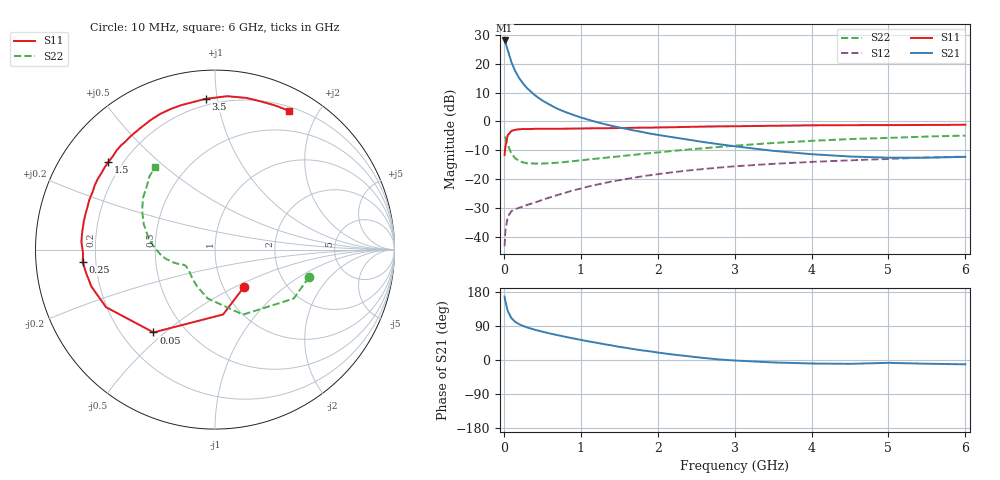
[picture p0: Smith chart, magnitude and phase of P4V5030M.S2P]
! SIEMENS Small Signal Semiconductors
! BFP182
! Si NPN RF Bipolar Junction Transistor in SOT143
! VCE = 0.5 V  IC = 30 mA
! Common Emitter S-Parameters:  March  1996
# GHz  S  MA  R  50
!  f  S11  S21  S12  S22
! GHz  MAG  ANG  MAG  ANG  MAG  ANG  MAG  ANG
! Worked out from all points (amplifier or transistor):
!   36 points, 10 MHz to 6 GHz, reference 50 ohm
!   highest |S21| = 28.2 dB at 10 MHz (marker M1)
!   |S21| within 3 dB of that: start of sweep to 46.69 MHz
!   unconditionally stable (mu >= 1): start of sweep to 23.08 MHz; 140.7 MHz to end of sweep
!   at 250 MHz: K = 1.46, MAG = 17.4 dB, |S12| = -29.6 dB
!   at 1.4 GHz: K = 2.64, MAG = 2.6 dB, |S12| = -20.9 dB
!   at 6 GHz: K = 1.82, MAG = -5.3 dB, |S12| = -12.2 dB
!   S11 on the Smith chart (normalised r, x): 10 MHz: 1.25, -0.56; 50 MHz: 0.33, -0.46; 250 MHz: 0.15, -0.05; 1.5 GHz: 0.15, +0.35; 3.5 GHz: 0.16, +0.93; 6 GHz: 0.25, +1.63
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0.01  0.2631 -51.7  25.61 167.1  0.0068 68.2  0.546 -16.3
0.02  0.3644 -82.9  24.13 155.2  0.0124 61.4  0.5161 -31.9
0.05  0.5747 -126.6  17.5 129.6  0.022 45.5  0.3944 -66.7
0.1  0.687 -152.2  10.62 110.0  0.0277 32.5  0.2752 -98.5
0.15  0.7189 -163.4  7.424 100.4  0.0299 31.1  0.2279 -116.1
0.2  0.7299 -169.8  5.663 94.4  0.0317 31.8  0.2058 -127.1
0.25  0.7405 -174.6  4.575 89.8  0.0333 33.0  0.1943 -134.1
0.3  0.7355 -178.2  3.822 86.1  0.0353 36.5  0.1881 -139.2
0.4  0.7457 176.5  2.881 80.0  0.039 39.9  0.1857 -146.1
0.5  0.7463 172.2  2.312 74.9  0.0433 42.4  0.1859 -149.6
0.6  0.7476 168.0  1.946 69.9  0.048 45.5  0.1878 -151.8
0.7  0.7484 164.5  1.657 65.5  0.0528 47.5  0.1923 -153.5
0.9  0.7535 158.3  1.306 57.1  0.0635 49.5  0.2047 -156.2
1.1  0.7598 152.0  1.073 49.2  0.0741 50.0  0.2185 -158.5
1.5  0.7691 140.6  0.787 34.6  0.0953 48.4  0.2472 -163.6
1.8  0.7817 132.2  0.657 25.3  0.1114 46.2  0.2735 -168.3
2.2  0.7939 122.0  0.531 14.4  0.1312 42.0  0.3084 -175.6
2.8  0.8216 107.3  0.402 1.4  0.1582 34.7  0.3611 173.0
3.5  0.8419 93.5  0.309 -6.4  0.1834 26.1  0.4226 160.1
4.5  0.8632 78.2  0.246 -10.1  0.2111 14.7  0.4948 144.1
5.5  0.8703 67.1  0.235 -9.8  0.237 4.5  0.5475 131.8
6  0.8762 62.1  0.243 -11.4  0.2443 -0.9  0.5683 126.0
